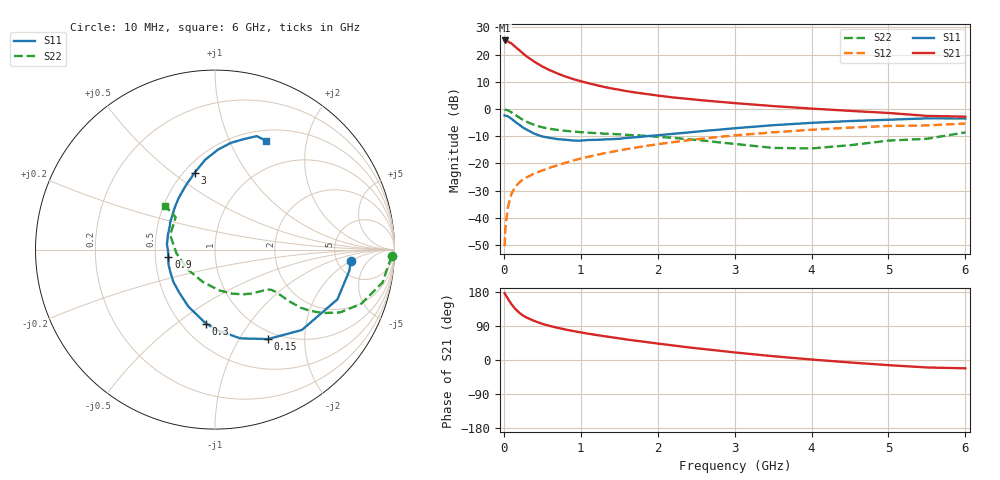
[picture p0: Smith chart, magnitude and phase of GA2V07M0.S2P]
! Infineon Technologies  Discrete & RF Semiconductors
! BF775
! Si NPN RF Bipolar Junction Transistor in SOT23
! VCE = 2 V  IC = 7 mA
! Common Emitter S-Parameters:  May  1996
# GHz  S  MA  R  50
!  f  S11  S21  S12  S22
! GHz  MAG  ANG  MAG  ANG  MAG  ANG  MAG  ANG
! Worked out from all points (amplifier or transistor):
!   36 points, 10 MHz to 6 GHz, reference 50 ohm
!   highest |S21| = 25.2 dB at 10 MHz (marker M1)
!   |S21| within 3 dB of that: start of sweep to 176.5 MHz
!   unconditionally stable (mu >= 1): 650.2 MHz to 3.784 GHz; 5.479 GHz to 5.542 GHz
!   at 250 MHz: K = 0.60, MSG = 23.2 dB, |S12| = -25.9 dB
!   at 1.4 GHz: K = 1.14, MAG = 9.4 dB, |S12| = -15.8 dB
!   at 6 GHz: K = 0.99, MSG = 1.3 dB, |S12| = -5.3 dB
!   S11 on the Smith chart (normalised r, x): 10 MHz: 6.73, -2.04; 150 MHz: 0.89, -1.34; 300 MHz: 0.65, -0.65; 900 MHz: 0.59, -0.05; 3 GHz: 0.56, +0.60; 6 GHz: 0.63, +1.38
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0.01  0.7608 -4.8  18.25 176.5  0.003 87.0  0.9854 -2.2
0.02  0.757 -9.2  17.99 172.6  0.0064 82.9  0.9731 -4.5
0.05  0.7363 -22.1  17.62 162.5  0.015 79.2  0.9513 -11.1
0.1  0.6594 -42.8  16.04 147.2  0.0279 70.1  0.8682 -20.4
0.15  0.5791 -59.4  13.87 134.4  0.0374 64.1  0.7793 -26.7
0.2  0.5146 -74.0  12.13 124.9  0.0445 60.8  0.6966 -30.5
0.25  0.4555 -86.6  10.53 117.2  0.0506 58.2  0.6282 -32.8
0.3  0.4157 -96.9  9.213 111.5  0.0557 57.7  0.5787 -34.1
0.4  0.3499 -115.2  7.37 102.7  0.0654 57.2  0.5087 -34.8
0.5  0.3124 -129.3  6.057 95.4  0.0741 58.0  0.4605 -34.8
0.6  0.2941 -141.8  5.16 89.8  0.0834 58.6  0.4317 -34.8
0.7  0.2794 -152.4  4.496 84.9  0.0927 59.3  0.4126 -34.8
0.9  0.2634 -170.6  3.559 76.5  0.1127 59.5  0.3849 -35.6
1.1  0.2696 173.8  2.983 69.4  0.1325 59.6  0.3673 -37.6
1.3  0.2751 162.2  2.555 63.0  0.1529 58.6  0.353 -40.0
1.6  0.2951 147.3  2.127 54.0  0.1837 56.7  0.3348 -44.8
2.2  0.3498 125.6  1.633 38.4  0.2457 51.3  0.2955 -57.6
3  0.4429 104.9  1.285 20.0  0.3269 41.9  0.2284 -84.1
3.5  0.5039 96.2  1.133 10.0  0.3724 35.4  0.1925 -110.5
4.5  0.601 81.6  0.925 -6.5  0.4554 22.1  0.216 -174.8
5.5  0.6734 69.8  0.748 -19.7  0.4988 7.7  0.2836 140.6
6  0.6695 64.9  0.723 -22.0  0.5406 3.6  0.3712 138.7
